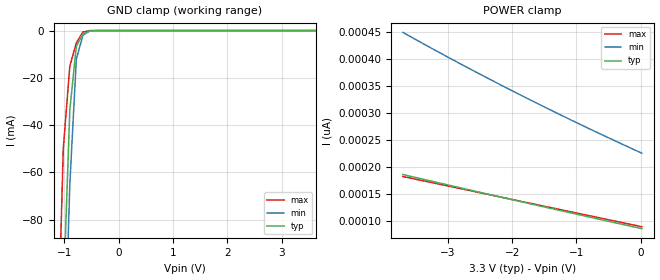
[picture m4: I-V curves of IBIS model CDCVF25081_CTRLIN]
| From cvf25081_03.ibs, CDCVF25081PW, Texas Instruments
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|   Model CDCVF25081_CTRLIN
[Model]   CDCVF25081_CTRLIN
Model_type   Input
Polarity   Non-Inverting
Vinl = 0.8V
Vinh = 2.0V
| variable   typ   min   max
C_comp   2.1pF   NA   NA
[Temperature Range]   40   85   -40
[Voltage range]   3.3   3.0   3.6
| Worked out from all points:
|   GND clamp passes 1 mA (typ) near -0.61 V on its own axis
|Process range|   nominal   weak   strong
[GND Clamp]
|   40C:3.3V:nominal   85C:3.0V:weak   -40C:3.6V:strong
|  Voltage   I(typ)   I(min)   I(max)
-3.66V    -2.664A    -2.705A    -2.597A
-1.26V    -322.3mA   -368mA     -246.9mA
-1.02V    -112.9mA   -155.7mA   -49.9mA
-900mV    -33.58mA   -65.08mA   -15.03mA
-780mV    -6.672mA   -12.13mA   -5.186mA
-660mV    -1.52mA    -2.065mA   -636uA
-540mV    -141uA     -274.6uA   -17.91uA
-420mV    -6.132uA   -20.13uA   -140.8nA
3.64V     95.43pA    262.2pA    91.01pA
[POWER Clamp]
|   40C:3.3V:nominal   85C:3.0V:weak   -40C:3.6V:strong
|  Voltage   I(typ)   I(min)   I(max)
-3.7V     186.2pA    449.5pA    182.5pA
-2.74V    159.7pA    387.2pA    158.5pA
-1.78V    133.8pA    328.2pA    134.5pA
-940mV    111.3pA    279.1pA    113.5pA
20mV      85.94pA    225.8pA    89.51pA
